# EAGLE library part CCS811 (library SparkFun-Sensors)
AMS CCS811 &ndash; I2C Digital Gas Sensor Ultra-Low Power Digital Gas Sensor for Monitoring Indoor Air Quality AMS Product Page SparkFun Products:
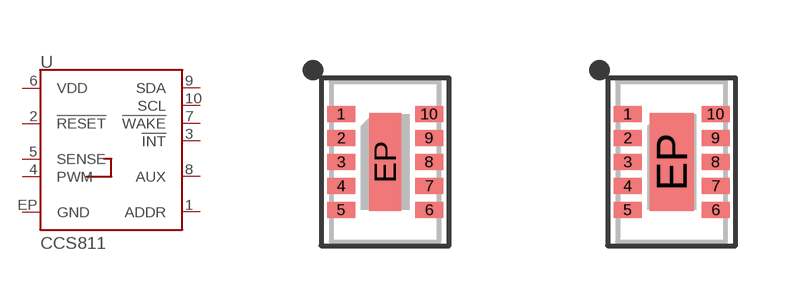
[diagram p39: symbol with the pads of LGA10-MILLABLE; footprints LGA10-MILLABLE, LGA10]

Designator prefix U

## CCS811SKINNY  [LGA10-MILLABLE]
1  ADDR
2  !RESET!
3  !INT!
4  PWM
5  SENSE
6  VDD
7  !WAKE!
8  AUX
9  SDA
10  SCL
EP  GND

## CCS811PRODUCTION (PROD_ID: IC-13607; VALUE: CCS811)  [LGA10]
Pads as for LGA10-MILLABLE

## Footprint LGA10-MILLABLE (pad centres in mm)
10-pin LGA package - 2.7 x 4.0mm, 0.6mm pitch Package specifications: Pin Count: 10 (+ exposed pad) Dimensions: 2.7mm x 4.0mm x 1.1mm Pitch: 0.6mm Used by: CCS811
smd 0.7 x 0.4: 1 -1.1,1.2; 2 -1.1,0.6; 3 -1.1,0; 4 -1.1,-0.6; 5 -1.1,-1.2; 6 1.1,-1.2; 7 1.1,-0.6; 8 1.1,0; 9 1.1,0.6; 10 1.1,1.2
smd 0.8 x 2.45: EP 0,0

## Footprint LGA10 (pad centres in mm)
smd 0.7 x 0.4: 1 -1.1,1.2; 2 -1.1,0.6; 3 -1.1,0; 4 -1.1,-0.6; 5 -1.1,-1.2; 6 1.1,-1.2; 7 1.1,-0.6; 8 1.1,0; 9 1.1,0.6; 10 1.1,1.2
smd 1.1 x 2.45: EP 0,0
